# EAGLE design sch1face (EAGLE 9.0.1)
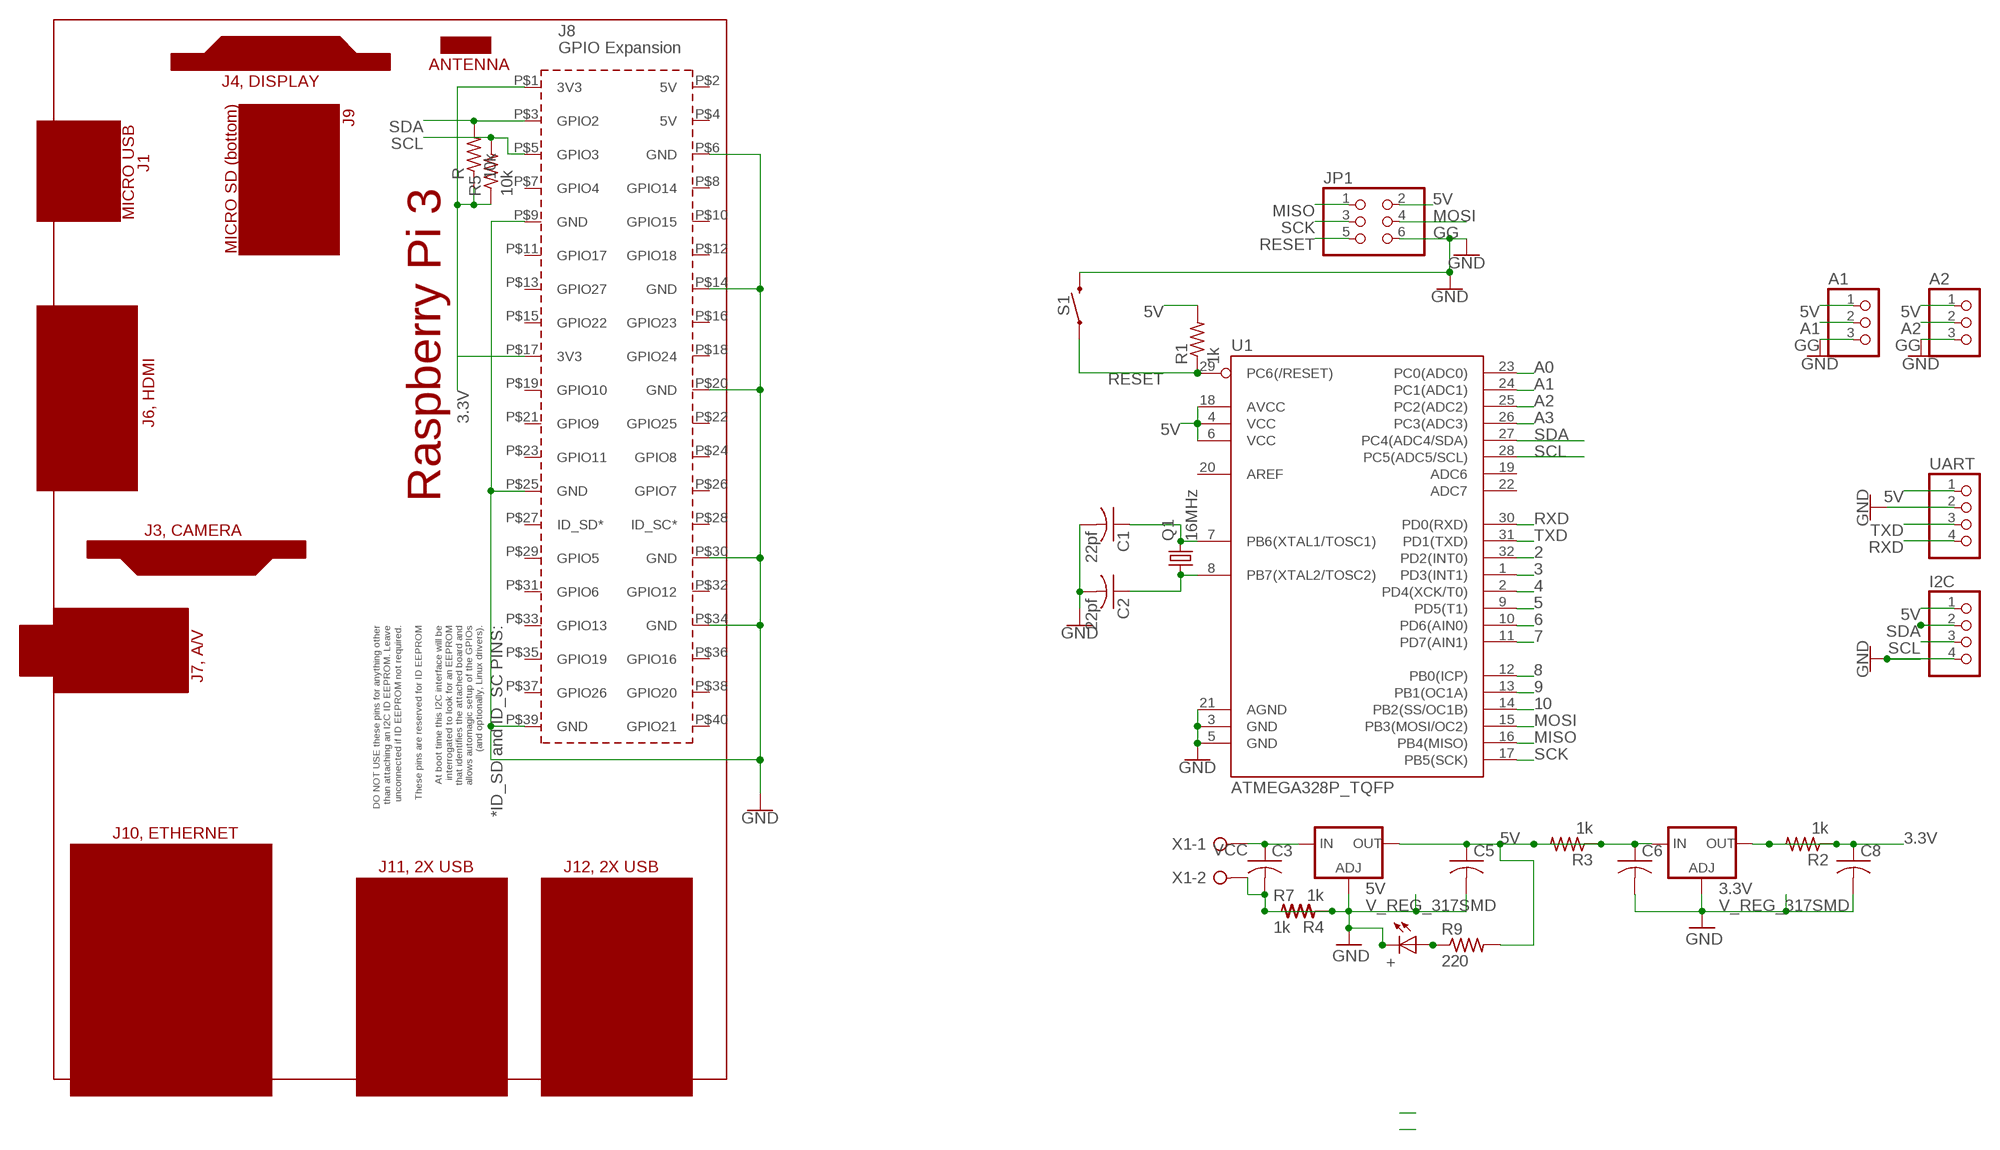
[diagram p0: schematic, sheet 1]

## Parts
3.3V  V_REG_317SMD  [SOT223]
5V  V_REG_317SMD  [SOT223]
+  LEDSML1206  [SML1206]
A1  PINHD-1X3  [1X03]
A2  PINHD-1X3  [1X03]
C1  22pf  C-USC1206  [C1206]
C2  22pf  C-USC1206  [C1206]
C3  C-USC1206  [C1206]
C5  C-USC1206  [C1206]
C6  C-USC1206  [C1206]
C8  C-USC1206  [C1206]
I2C  PINHD-1X4  [1X04]
JP1  PINHD-2X3  [2X03]
PCB1  RPI3  [RPI3]
Q1  16MHz  CRYSTALHC49UP  [HC49UP]
R  10k  R-US_M1206  [M1206]
R1  1k  R-US_M1206  [M1206]
R2  1k  R-US_M1206  [M1206]
R3  1k  R-US_M1206  [M1206]
R4  1k  R-US_M1206  [M1206]
R5  10k  R-US_M1206  [M1206]
R7  1k  R-US_M1206  [M1206]
R9  220  R-US_M1206  [M1206]
S1  MOMENTARY-SWITCH-SPST-SMD-6.2MM-TALL  [TACTILE_SWITCH_SMD_6.2MM_TALL]
U1  ATMEGA328P_TQFP  [TQFP32-08]
UART  PINHD-1X4  [1X04]
X1  W237-02P  [W237-132]

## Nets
2: U1.32(PD2(INT0))
3: U1.1(PD3(INT1))
3.3V: 3.3V.2(OUT) C8.1 PCB1.P$1(3V3) PCB1.P$17(3V3) R2.1 R2.2 R5.1 R.1
4: U1.2(PD4(XCK/T0))
5: U1.9(PD5(T1))
5V: 3.3V.3(IN) 5V.2(OUT) A1.1 A2.1 C5.1 C6.1 I2C.1 JP1.2 R1.2 R3.1 R3.2 R9.2 U1.4(VCC) U1.6(VCC) U1.18(AVCC) UART.1
6: U1.10(PD6(AIN0))
7: U1.11(PD7(AIN1))
8: U1.12(PB0(ICP))
9: U1.13(PB1(OC1A))
10: U1.14(PB2(SS/OC1B))
A0: U1.23(PC0(ADC0))
A1: A1.2 U1.24(PC1(ADC1))
A2: A2.2 U1.25(PC2(ADC2))
A3: U1.26(PC3(ADC3))
GG: 3.3V.1(ADJ) 5V.1(ADJ) +.C A1.3 A2.3 C1.2 C2.2 C3.2 C5.2 C6.2 C8.2 I2C.4 JP1.6 PCB1.P$6(GND) PCB1.P$9(GND) PCB1.P$14(GND) PCB1.P$20(GND) PCB1.P$25(GND) PCB1.P$30(GND) PCB1.P$34(GND) PCB1.P$39(GND) R4.1 R4.2 R7.1 R7.2 S1.B2 U1.3(GND) U1.5(GND) U1.21(AGND) UART.2 X1.2 ; supply symbol labelled GND
MISO: JP1.1 U1.16(PB4(MISO))
MOSI: JP1.4 U1.15(PB3(MOSI/OC2))
N$1: C1.1 Q1.2 U1.7(PB6(XTAL1/TOSC1))
N$2: C2.1 Q1.1 U1.8(PB7(XTAL2/TOSC2))
N$4: +.A R9.1
RESET: JP1.5 R1.1 S1.A2 U1.29(PC6(/RESET))
RXD: U1.30(PD0(RXD)) UART.4
SCK: JP1.3 U1.17(PB5(SCK))
SCL: I2C.3 PCB1.P$5(GPIO3) R5.2 U1.28(PC5(ADC5/SCL))
SDA: I2C.2 PCB1.P$3(GPIO2) R.2 U1.27(PC4(ADC4/SDA))
TXD: U1.31(PD1(TXD)) UART.3
VCC: 5V.3(IN) C3.1 X1.1
Unconnected: PCB1.P$2(5V) PCB1.P$4(5V) PCB1.P$7(GPIO4) PCB1.P$8(GPIO14) PCB1.P$10(GPIO15) PCB1.P$11(GPIO17) PCB1.P$12(GPIO18) PCB1.P$13(GPIO27) PCB1.P$15(GPIO22) PCB1.P$16(GPIO23) PCB1.P$18(GPIO24) PCB1.P$19(GPIO10) PCB1.P$21(GPIO9) PCB1.P$22(GPIO25) PCB1.P$23(GPIO11) PCB1.P$24(GPIO8) PCB1.P$26(GPIO7) PCB1.P$27(ID_SD*) PCB1.P$28(ID_SC*) PCB1.P$29(GPIO5) PCB1.P$31(GPIO6) PCB1.P$32(GPIO12) PCB1.P$33(GPIO13) PCB1.P$35(GPIO19) PCB1.P$36(GPIO16) PCB1.P$37(GPIO26) PCB1.P$38(GPIO20) PCB1.P$40(GPIO21) U1.19(ADC6) U1.20(AREF) U1.22(ADC7)

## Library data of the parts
3.3V 5V = SparkFun-IC-Power:V_REG_317: Voltage Regulator Standard LM317 adjustable voltage regulator. AOI (Adjust Output Input). Google 'LM317 Calculator' for easy to use app to get the two resistor values needed. 240/720 for 5V output. 240/390 for 3.3V output. Spark Fun Electronics SKU : COM-00527
+ = led:LED: LED
A1 A2 = pinhead:PINHD-1X3: PIN HEADER
C1 C2 = rcl:C-US: CAPACITOR, American symbol
C3 C5 C6 C8 = resistor:C-US: CAPACITOR, American symbol
I2C UART = pinhead:PINHD-1X4: PIN HEADER
JP1 = pinhead:PINHD-2X3: PIN HEADER
PCB1 = e14_Rpi3_RevA:RPI3: Device for Raspberry Pi 3 board created by Dave Young for www.element14.com More information and support community is available at https://www.element14.com/community/community/raspberry-pi
Q1 = crystal:CRYSTAL: CRYSTAL; OC_FARNELL: unknown; OC_NEWARK: unknown
R R1-R5 R7 R9 = resistor:R-US_: RESISTOR, American symbol
S1 = SparkFun-Switches:MOMENTARY-SWITCH-SPST: Momentary Switch (Pushbutton) - SPST; PROD_ID: SWCH-11966; SF_SKU: COM-12992
U1 = SparkFun-DigitalIC:ATMEGA328P_TQFP; PROD_ID: IC-09069
X1 = con-wago-508:W237-02P: WAGO SREW CLAMP; OC_FARNELL: unknown; OC_NEWARK: unknown

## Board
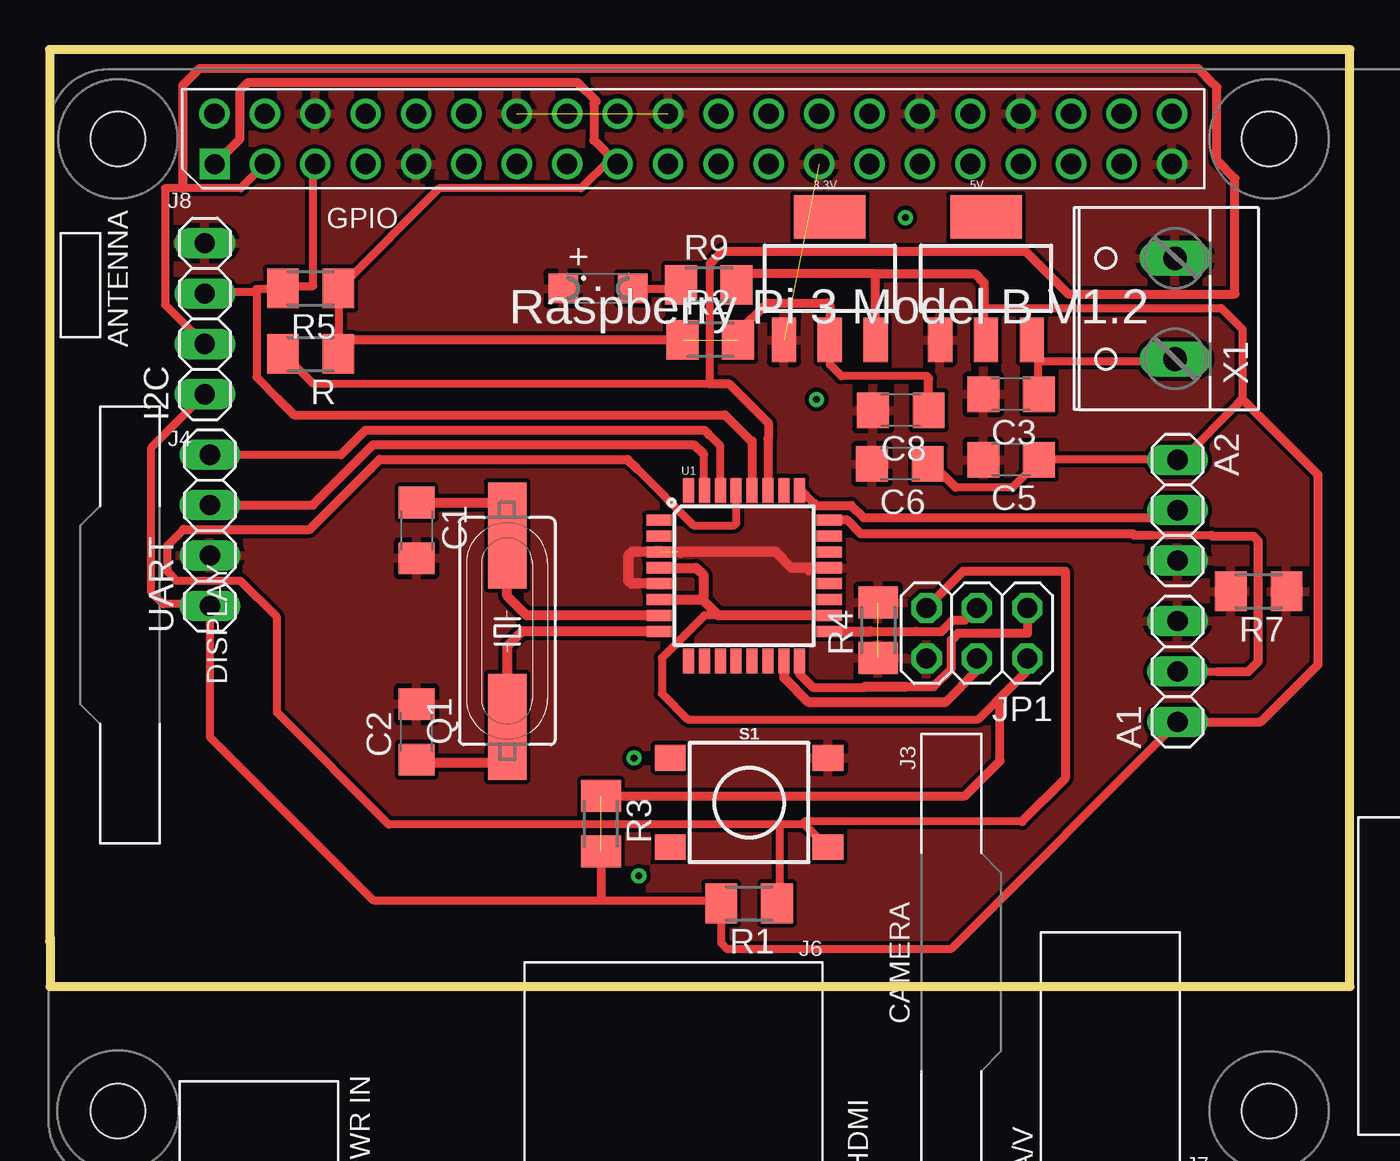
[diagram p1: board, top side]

Size 65.53 x 47.22 mm. Coordinates in mm from the lower left corner, seen from the top.
Outline: 0.03,2.49 0.03,0 65.53,0 65.53,47.22 0,47.22 0,2.29
Copper layers (1*16): Top 0.035mm / dielectric 1.5mm / Bottom 0.035mm
Design rules "default *": minimum track width 16mil, minimum drill 0.35mm, track to track 8mil, track to pad 8mil, pad to pad 8mil, via to via 8mil, smd to smd 6mil, copper to edge 40mil, drill to drill 6mil, minimum pad ring 10mil, minimum via ring 8mil, stop-mask expansion 4mil, vias tented up to drill 0mil, thermal gap 10mil

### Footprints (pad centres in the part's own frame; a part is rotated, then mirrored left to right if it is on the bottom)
SOT223 = smd 1.219 x 2.235: 1 -2.311,-3.099; 2 0,-3.099; 3 2.311,-3.099 | smd 3.6 x 2.2: 4 0,3.099
SML1206 = smd 1.5 x 1.5: A 1.75,0; C -1.75,0
1X03 = drill 1.016 long: 1 -2.54,0; 2 0,0; 3 2.54,0
C1206 = smd 1.6 x 1.8: 1 -1.4,0; 2 1.4,0
1X04 = drill 1.016 long: 1 -3.81,0; 2 -1.27,0; 3 1.27,0; 4 3.81,0
2X03 = drill 1.016 octagon: 1 -2.54,-1.27; 2 -2.54,1.27; 3 0,-1.27; 4 0,1.27; 5 2.54,-1.27; 6 2.54,1.27
RPI3 = drill 1.016 square: P$1 8.37,51.23 | drill 1.016: P$2 8.357,53.772; P$3 10.897,51.232; P$4 10.897,53.772; P$5 13.437,51.232; P$6 13.437,53.772; P$7 15.977,51.232; P$8 15.977,53.772; P$9 18.517,51.232; P$10 18.517,53.772; P$11 21.057,51.232; P$12 21.057,53.772; P$13 23.597,51.232; P$14 23.597,53.772; P$15 26.137,51.232; P$16 26.137,53.772; P$17 28.677,51.232; P$18 28.677,53.772; P$19 31.217,51.232; P$20 31.217,53.772; P$21 33.757,51.232; P$22 33.757,53.772; P$23 36.297,51.232; P$24 36.297,53.772; P$25 38.837,51.232; P$26 38.837,53.772; P$27 41.377,51.232; P$28 41.377,53.772; P$29 43.917,51.232; P$30 43.917,53.772; P$31 46.457,51.232; P$32 46.457,53.772; P$33 48.997,51.232; P$34 48.997,53.772; P$35 51.537,51.232; P$36 51.537,53.772; P$37 54.077,51.232; P$38 54.077,53.772; P$39 56.617,51.232; P$40 56.617,53.772 | hole 2.75: 3.5,3.5; 61.5,3.5; 3.5,52.5; 61.5,52.5
HC49UP = smd 5.334 x 1.93: 1 -4.826,0; 2 4.826,0
M1206 = smd 1.6 x 2: 1 -1.4,0; 2 1.4,0
TACTILE_SWITCH_SMD_6.2MM_TALL = smd 1.55 x 1.3: A1 -3.975,-2.25; A2 3.975,-2.25; B1 -3.975,2.25; B2 3.975,2.25
TQFP32-08 = smd 1.27 x 0.559: 1 -4.293,2.8; 2 -4.293,2; 3 -4.293,1.2; 4 -4.293,0.4; 5 -4.293,-0.4; 6 -4.293,-1.2; 7 -4.293,-2; 8 -4.293,-2.8; 17 4.293,-2.8; 18 4.293,-2; 19 4.293,-1.2; 20 4.293,-0.4; 21 4.293,0.4; 22 4.293,1.2; 23 4.293,2; 24 4.293,2.8 | smd 0.559 x 1.27: 9 -2.8,-4.293; 10 -2,-4.293; 11 -1.2,-4.293; 12 -0.4,-4.293; 13 0.4,-4.293; 14 1.2,-4.293; 15 2,-4.293; 16 2.8,-4.293; 25 2.8,4.293; 26 2,4.293; 27 1.2,4.293; 28 0.4,4.293; 29 -0.4,4.293; 30 -1.2,4.293; 31 -2,4.293; 32 -2.8,4.293
W237-132 = drill 1.194 long: 1 -2.54,-0.635; 2 2.54,-0.635

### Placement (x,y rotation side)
3.3V  39.32,35.69 0 top
5V  47.19,35.69 0 top
+  27.64,35.18 0 top
A1  56.85,15.88 90 top
A2  56.85,24 270 top
C1  18.49,22.99 270 top
C2  18.49,12.83 90 top
C3  48.46,29.85 180 top
C5  48.46,26.54 180 top
C6  42.85,26.34 180 top
C8  42.9,29.03 180 top
I2C  7.82,33.66 90 top
JP1  46.74,17.81 180 top
PCB1  -0.05,-9.78 0 top
Q1  23.06,17.91 90 top
R  13.16,31.88 180 top
R1  35.26,4.19 180 top
R2  33.3,32.59 0 top
R3  27.79,8.2 270 top
R4  41.76,17.96 90 top
R5  13.16,35.18 180 top
R7  60.93,19.91 180 top
R9  33.22,35.36 0 top
S1  35.26,9.27 0 top
U1  35,20.7 0 top
UART  8.08,22.99 90 top
X1  56.08,34.16 90 top

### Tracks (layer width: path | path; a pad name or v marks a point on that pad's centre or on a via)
3.3V  (1 unrouted)
  Top 0.406: R.1 14.55,31.97 14.55,32.18 14.55,35.15 R5.1 14.71,35.31 19.63,40.23 26.78,40.23 28.21,41.66 PCB1.P$17 28.52,41.5 | 8.36,41.5 PCB1.P$1 | 3.3V.2 39.32,31.34 39.9,30.76 44.2,30.76
  Top 0.457: C8.1 44.3,30.65 44.2,30.76 | 3.3V.2 39.32,34.34 39.22,34.44 36.17,34.44 34.7,32.97 R2.2 34.7,33.15 | 14.55,32.18 14.96,32.59 R2.1 | PCB1.P$1 9.6,42.73 9.6,45.16 10.01,45.57 26.59,45.57 27.55,44.61 27.43,44.49 27.43,42.65 PCB1.P$17
5V  (1 unrouted)
  Top 0.406: 45.67,25.15 48.53,25.15 49.8,26.42 C5.1 49.96,26.57 56.78,26.57 A2.1 56.94,26.42 60.12,29.6 60.12,33.12 59.05,34.19 47.1,34.19 47.1,32.61 5V.2 | 44.4,26.42 C6.1 44.24,26.73 | 34.72,35.15 R9.2 | 41.7,32.61 3.3V.3 41.7,32.45 | UART.1 8.05,19.27 5.72,19.27 5.13,19.86 5.13,27.15 I2C.1 | R1.2 33.92,4.19 | 56.78,13.24 A1.1 56.94,13.4 45.42,1.88 34.16,1.88 33.86,2.19 R1.2 | 8.2,19.11 UART.1 | R1.2 33.76,4.35 27.79,4.35 16.3,4.35 8.08,12.57 UART.1 | 33.7,18.7 33,18.7 30.86,16.56 30.86,14.76 32.16,13.46 46.81,13.46 47.7,14.35
  Top 0.457: R9.2 | R9.2 35.18,35.18 | 41.61,35.92 46.63,35.92 47.1,35.45 47.1,34.19 | 3.3V.3 41.63,35.89 41.61,35.92 | 45.67,25.15 44.4,26.42 | R9.2 35.18,35.92 41.61,35.92 | R3.2 27.79,4.35 | R3.1 46.13,9.6 47.9,11.38 47.9,14.15 47.7,14.35 49.28,15.93 JP1.2 | 59.84,29.32 60.12,29.6 63.93,25.79 63.93,16.23 61.04,13.34 A1.1
  Top 0.508: U1.4 32.57,21.1 32.97,20.7 32.97,19.68 32.84,19.56 | U1.6 32.79,19.5 32.84,19.56 | U1.18 33.7,18.7 32.84,19.56
A1
  Top 0.406: U1.24 39.32,23.56 | 58.57,22.73 55.55,22.73 | A1.2 58.88,15.88
  Top 0.457: 55.55,22.73 54.66,22.73 54.58,22.81 40.9,22.81 40.21,23.5 U1.24 | 58.88,15.88 60.4,15.88 60.91,16.38 60.91,22.45 60.68,22.68 58.62,22.68 58.57,22.73
A2
  Top 0.406: 38.53,24.35 37.89,24.99 U1.25 | 56.46,24.35 56.78,24.04 A2.2
  Top 0.457: 38.53,24.35 38.63,24.25 40.4,24.25 41.02,23.62 56.46,23.62 A2.2
GG  (4 unrouted)
  Top 0.406: 38.25,20.93 38.2,21.1 | 31.65,21.92 31.8,21.81
  Top 0.508: U1.5 29.31,20.3 29.16,20.45 29.16,21.72 29.34,21.9 U1.3 36.6,21.9 37.4,21.1 U1.21
  pour Top: 3.63,47.6 65.81,47.6 65.81,0.28 0,0.28 0,47.57 3.68,47.57
MISO
  Top 0.457: 43.15,15.11 44.55,15.11 45.44,16 45.44,17.45 45.8,17.8 49.3,17.8 49.3,19.05 JP1.1 | U1.16 37.8,15.75 38.47,15.08 41.06,15.08 41.1,15.11
  Top 0.508: 41.1,15.11 43.15,15.11
MOSI
  Top 0.457: 45.16,14.35 46.74,15.93 JP1.4
  Top 0.508: U1.15 37.01,16.4 37.01,15.56 38.23,14.35 45.16,14.35
N$1
  Top 0.508: U1.7 24.05,18.7 23.06,19.68 Q1.2 23.06,24 22.68,24.39 C1.1
N$2
  Top 0.508: U1.8 23.82,17.9 23.06,17.14 Q1.1 23.06,11.3 18.62,11.3 C2.1
N$4
  Top 0.406: +.A 29.48,35.15 31.7,35.15 R9.1
N$6  (via drill 0.35)
  other vias: 38.66,29.59
N$7  (via drill 0.35)
  other vias: 43.13,38.76
N$8  (via drill 0.35)
  other vias: 29.69,5.56
N$9  (via drill 0.35)
  other vias: 29.46,11.51
RESET
  Top 0.406: 38.05,8.16 36.78,8.16 | 36.78,8.16 17.09,8.16 11.46,13.8 11.46,18.62 9.63,20.45 6.4,20.45 5.94,20.9 5.94,22.22 6.76,23.04 | 38.05,8.16 39.16,7.05 S1.A2 | 34.56,25.15 U1.29 34.6,23.35 34.49,23.24 32.46,23.24 29.6,26.1 | 36.78,8.16 36.78,4.19 R1.1 | 49,8.32 38.05,8.32 38.05,8.16
  Top 0.457: 6.76,23.04 13.11,23.04 16.18,26.11 | 16.18,26.11 16.19,26.1 | 16.18,26.11 16.64,26.57 29.13,26.57 29.6,26.1 | JP1.5 46.05,20.93 51.18,20.93 51.18,10.5 49,8.32
RXD
  Top 0.406: UART.4 14.68,26.8 | U1.30 33.8,27.24 33.22,27.81
  Top 0.457: 14.68,26.8 15.93,28.04 32.99,28.04 33.22,27.81
SCK
  Top 0.457: 41.36,17.9 43.68,17.9 43.7,17.88 44.94,17.88 45.52,18.47 46.13,18.47 JP1.3
  Top 0.508: U1.17 41.36,17.9
SCL
  Top 0.406: 11.54,29.59 10.43,30.7 10.43,34.99 | 10.43,34.99 10.43,35.15 11.7,35.15 R5.2 11.86,35.31 13.28,35.31 13.28,41.34 PCB1.P$5 | 35.4,25.15 U1.28 | 10.43,34.99 7.89,34.99 I2C.3
  Top 0.457: 11.54,29.59 12.33,28.8 34.04,28.8 35.4,27.44 | 35.4,27.49 35.4,27.44 | 35.4,25.15 35.4,27.43 35.4,27.44
SDA
  Top 0.406: I2C.2 7.73,32.45 5.82,34.35 5.82,40.23 6.68,40.23 9.63,40.23 10.74,41.34 PCB1.P$3 | 36.14,25.15 U1.27 | R.2 11.86,31.81 13.28,30.39 33.29,30.39 33.29,36.42
  Top 0.457: U1.27 36.2,27.59 36.22,27.61 36.22,28.4 34.23,30.39 33.29,30.39 | 33.29,36.42 33.39,36.52 33.39,36.54 33.92,37.06 49.17,37.06 51.33,34.9 59.74,34.9 59.74,40.72 58.83,41.64 58.83,45.31 58.48,45.66 58.32,45.82 57.86,46.28 7.57,46.28 6.73,45.44 6.73,40.28 6.68,40.23
TXD
  Top 0.406: U1.31 32.97,25.03 32.97,26.8
  Top 0.457: 32.97,26.8 32.46,27.31 16.31,27.31 13.26,24.26 UART.3
VCC
  Top 0.406: C3.1 49.8,29.91 49.8,32.45 49.64,32.45 5V.3 49.96,31.5 56.62,31.5 X1.1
